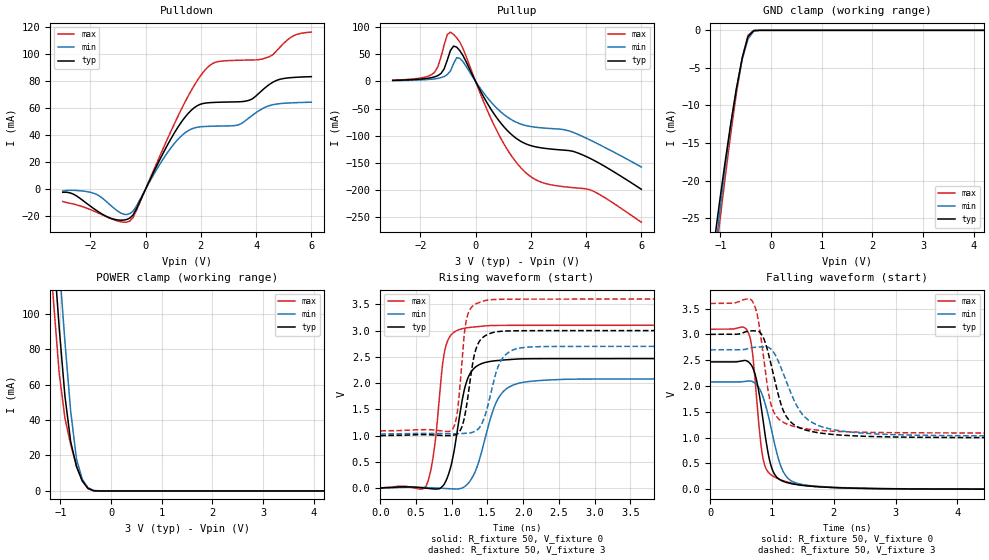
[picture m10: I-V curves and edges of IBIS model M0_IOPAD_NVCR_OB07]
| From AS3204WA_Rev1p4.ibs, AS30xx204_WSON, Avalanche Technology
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[Model] M0_IOPAD_NVCR_OB07
Model_type I/O
Enable   Active-High
Vinl  =  0.9
Vinh  =  2.1
Vmeas =  1.5
Cref  =  30e-12
| Capacitance  typ   min   max
C_comp   3.872127e-12   3.590660e-12   4.176448e-12
| Variables   typ   min   max
[GND Clamp Reference]   0   0   0
[POWER Clamp Reference]   3   2.7   3.6
[Pulldown Reference]   0   0   0
[Pullup Reference]   3   2.7   3.6
[Temperature Range]   25   105   -40
[Voltage Range]   3   2.7   3.6
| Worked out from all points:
|   slope of the pulldown table from 0 to 0.45 V, typ, clamps not added: 23.6 ohm
|   slope of the pullup table from 0 to 0.45 V, typ, clamps not added: 10.6 ohm
|   GND clamp passes 1 mA (typ) near -0.46 V on its own axis
|   POWER clamp passes 1 mA (typ) near -0.42 V on its own axis
|   falling waveform, R_fixture 50, V_fixture 0: 20-80 % time 201ps typ, 266ps min, 152ps max; typ from 2.47 V to 0 V
|   falling waveform, R_fixture 50, V_fixture 3: 20-80 % time 290ps typ, 421ps min, 196ps max; typ from 3 V to 0.999 V
|   rising waveform, R_fixture 50, V_fixture 0: 20-80 % time 194ps typ, 277ps min, 142ps max; typ from 0 V to 2.47 V
|   rising waveform, R_fixture 50, V_fixture 3: 20-80 % time 142ps typ, 205ps min, 100ps max; typ from 0.999 V to 3 V
[GND Clamp]
| Voltage   I(typ)   I(min)   I(max)
-3V       -145.9mA   -151.9mA   -144.2mA
-1.138V   -29.07mA   -31.55mA   -32.68mA
-1.024V   -23.24mA   -24.83mA   -26.15mA
-910.3mV  -17.69mA   -18.46mA   -19.83mA
-796.6mV  -12.47mA   -12.67mA   -13.82mA
-682.8mV  -7.718mA   -7.754mA   -8.316mA
-569mV    -3.663mA   -3.867mA   -3.675mA
-455.2mV  -839.2uA   -1.152mA   -666.1uA
-341.4mV  -35.63uA   -111.1uA   -11.17uA
-113.8mV  -8.642nA   -188.3nA   -1.888nA
6V        0A         0A         0A
[POWER Clamp]
| Voltage   I(typ)   I(min)   I(max)
-3V       949.8mA    984.2mA    923.5mA
-1.252V   183.6mA    221.4mA    154mA
-1.138V   136.7mA    174.2mA    107.6mA
-1.024V   92.09mA    128.1mA    66.35mA
-910.3mV  53.33mA    83.97mA    41.06mA
-796.6mV  27.72mA    44.75mA    25.94mA
-682.8mV  13.75mA    18.06mA    14.29mA
-569mV    5.664mA    6.605mA    5.738mA
-455.2mV  1.446mA    1.789mA    1.305mA
-341.4mV  77.09uA    287.6uA    62.73uA
-227.6mV  1.148uA    12.92uA    332nA
6V        0A         0A         0A
[Pulldown]
| Voltage   I(typ)   I(min)   I(max)
-3V       -2.369mA   -1.449mA   -9.112mA
-1.934V   -13.55mA   -2.695mA   -15.7mA
-1.138V   -22.31mA   -14.22mA   -22.73mA
-569mV    -21.4mA    -18.11mA   -23.59mA
1.138V    44.69mA    36mA       52.38mA
1.655V    58.29mA    44.37mA    72.96mA
2.172V    63.6mA     46.29mA    88.47mA
3.372V    64.51mA    47.51mA    95.24mA
3.869V    66.73mA    54.6mA     95.46mA
4.366V    75.55mA    60.8mA     97.04mA
5.359V    82.53mA    63.82mA    113.4mA
6V        83.11mA    64.24mA    116.1mA
[Pullup]
| Voltage   I(typ)   I(min)   I(max)
-3V       1.852mA    1.381mA    2.173mA
-1.479V   8.502mA    4.75mA     17.23mA
-1.138V   23mA       8.991mA    67.38mA
-910.3mV  57.09mA    19.31mA    91.01mA
-682.8mV  63.21mA    43.83mA    80.43mA
-569mV    56.67mA    42.61mA    72.17mA
724.1mV   -64.02mA   -47.13mA   -86.41mA
1.759V    -113.8mA   -80.67mA   -165.6mA
2.483V    -123.4mA   -86.07mA   -187.7mA
3.745V    -132.9mA   -98.56mA   -197mA
4.366V    -147.8mA   -113.7mA   -205.2mA
6V        -199mA     -158mA     -259.8mA
[Ramp]
dV/dt_r   1.4802/0.19387n  1.24755/0.276663n  1.86079/0.142013n
dV/dt_f   1.2009/0.289582n  1.00246/0.420947n  1.5071/0.195569n
R_load = 50
[Falling Waveform]
R_fixture = 50
V_fixture = 0
V_fixture_min = 0
V_fixture_max = 0
| Time   V(typ)   V(min)   V(max)
0s        2.467V     2.079V     3.101V
597.5ps   2.482V     2.095V     3.078V
671.2ps   2.391V     2.091V     2.761V
748.6ps   2.115V     2.027V     1.781V
825.7ps   1.58V      1.875V     809mV
889.9ps   1.031V     1.648V     432.2mV
998.3ps   398.6mV    1.107V     264.9mV
1.165ns   159.4mV    377.9mV    170mV
1.518ns   69.13mV    84.13mV    73.8mV
21.88ns   1.03uV     1.085uV    12.78uV
[Falling Waveform]
R_fixture = 50
V_fixture = 3
V_fixture_min = 2.7
V_fixture_max = 3.6
| Time   V(typ)   V(min)   V(max)
0s        3V         2.7V       3.6V
671.7ps   3.068V     2.741V     3.659V
762.6ps   3.066V     2.754V     3.366V
854.8ps   2.947V     2.758V     2.625V
950.9ps   2.581V     2.744V     1.807V
1.04ns    2.132V     2.628V     1.468V
1.272ns   1.344V     1.958V     1.247V
1.486ns   1.169V     1.456V     1.181V
1.756ns   1.092V     1.231V     1.141V
21.88ns   998.5mV    1.029V     1.088V
[Rising Waveform]
R_fixture = 50
V_fixture = 0
V_fixture_min = 0
V_fixture_max = 0
| Time   V(typ)   V(min)   V(max)
0s        479.4nV    484.7nV    12.17uV
637.2ps   -181.3uV   12.48mV    33.92mV
757.3ps   -18.6mV    5.263mV    760.1mV
877.8ps   43.21mV    -3.7mV     2.419V
1ns       483.4mV    -13.07mV   2.932V
1.172ns   1.848V     21.46mV    3.044V
1.288ns   2.245V     203.4mV    3.066V
1.688ns   2.436V     1.786V     3.099V
2.251ns   2.466V     2.051V     3.1V
21.88ns   2.467V     2.079V     3.101V
[Rising Waveform]
R_fixture = 50
V_fixture = 3
V_fixture_min = 2.7
V_fixture_max = 3.6
| Time   V(typ)   V(min)   V(max)
0s        998.5mV    1.029V     1.088V
1.007ns   1.005V     1.035V     1.113V
1.085ns   1.044V     1.036V     1.514V
1.172ns   1.311V     1.042V     2.889V
1.22ns    1.675V     1.047V     3.281V
1.338ns   2.645V     1.091V     3.508V
1.532ns   2.943V     1.718V     3.586V
1.729ns   2.99V      2.503V     3.597V
2.167ns   2.999V     2.692V     3.599V
21.88ns   3V         2.7V       3.6V
